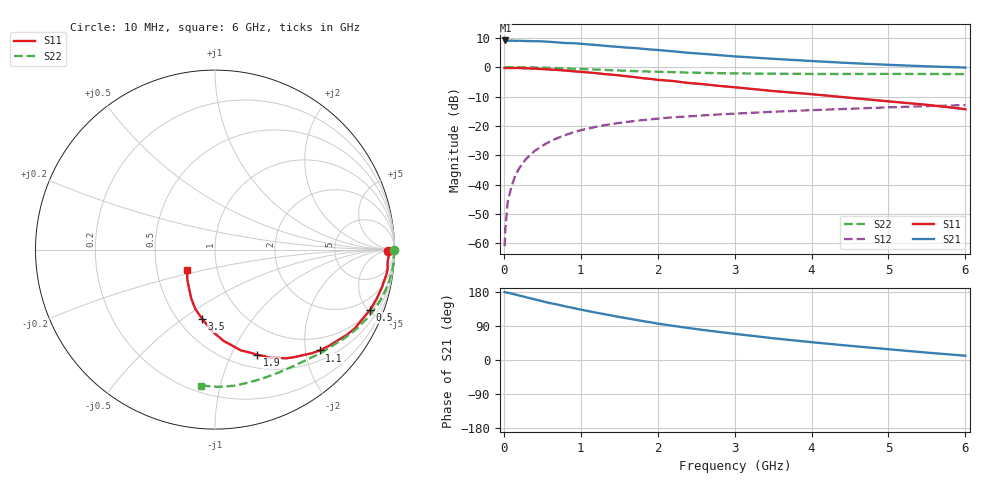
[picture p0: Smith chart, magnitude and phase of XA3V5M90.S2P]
! SIEMENS Discrete & RF Semiconductors
! BFY180
! Si NPN RF Bipolar Junction Transistor in MICRO-X
! VCE = 3.5 V  IC = 0.9 mA
! Common Emitter S-Parameters:  May  1997
# GHz  S  MA  R  50
!  f  S11  S21  S12  S22
! GHz  MAG  ANG  MAG  ANG  MAG  ANG  MAG  ANG
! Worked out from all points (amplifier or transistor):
!   36 points, 10 MHz to 6 GHz, reference 50 ohm
!   highest |S21| = 9.1 dB at 20 MHz (marker M1)
!   |S21| within 3 dB of that: start of sweep to 1.878 GHz
!   unconditionally stable (mu >= 1): 4.109 GHz to end of sweep
!   at 250 MHz: K = 0.07, MSG = 20.7 dB, |S12| = -32.5 dB
!   at 1.4 GHz: K = 0.48, MSG = 13.2 dB, |S12| = -19.4 dB
!   at 6 GHz: K = 1.05, MAG = 5.0 dB, |S12| = -12.9 dB
!   S11 on the Smith chart (normalised r, x): 10 MHz: 55, -11; 500 MHz: 1.06, -5.10; 1.1 GHz: 0.70, -2.30; 1.9 GHz: 0.65, -1.26; 3.5 GHz: 0.65, -0.59; 6 GHz: 0.71, -0.17
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0.01  0.9659 -0.4  2.82 179.5  0.0009 76.6  0.9962 -0.2
0.02  0.9637 -0.9  2.842 178.9  0.0018 89.0  0.9999 -0.6
0.05  0.9684 -2.2  2.802 177.6  0.0051 84.8  0.9979 -1.2
0.1  0.964 -4.1  2.826 175.3  0.0094 86.7  0.9967 -2.6
0.15  0.9678 -6.6  2.796 172.8  0.0145 85.7  0.9974 -3.9
0.25  0.9572 -10.8  2.792 167.8  0.0238 82.8  0.9948 -6.6
0.3  0.9539 -12.7  2.779 165.1  0.0283 80.9  0.9908 -7.8
0.5  0.9272 -21.3  2.747 155.1  0.0459 74.8  0.979 -12.8
0.6  0.9097 -24.8  2.69 150.1  0.0544 72.0  0.9709 -15.2
0.9  0.8505 -36.5  2.552 137.3  0.0775 63.9  0.941 -22.1
1.1  0.8103 -43.9  2.435 128.9  0.0902 59.0  0.9175 -26.3
1.5  0.7232 -56.9  2.207 113.5  0.1124 50.8  0.8762 -33.9
1.7  0.6767 -63.0  2.114 106.5  0.1209 47.3  0.8551 -37.3
1.9  0.6318 -68.1  2 99.8  0.1289 44.1  0.8398 -40.5
2.2  0.5799 -75.6  1.857 90.2  0.1402 40.0  0.8213 -45.2
2.6  0.5118 -84.5  1.68 79.0  0.1512 35.4  0.7976 -50.7
2.8  0.4791 -88.5  1.599 74.0  0.1568 33.4  0.7891 -53.3
3.5  0.392 -100.6  1.385 57.4  0.174 27.1  0.7717 -62.3
4  0.3465 -108.7  1.27 47.0  0.1852 22.9  0.7659 -68.7
4.5  0.3012 -116.2  1.172 37.4  0.1958 19.1  0.7642 -75.2
5.5  0.2285 -132.4  1.032 19.5  0.2169 11.2  0.765 -89.0
6  0.1924 -143.8  0.983 11.3  0.2256 7.0  0.7613 -95.9
